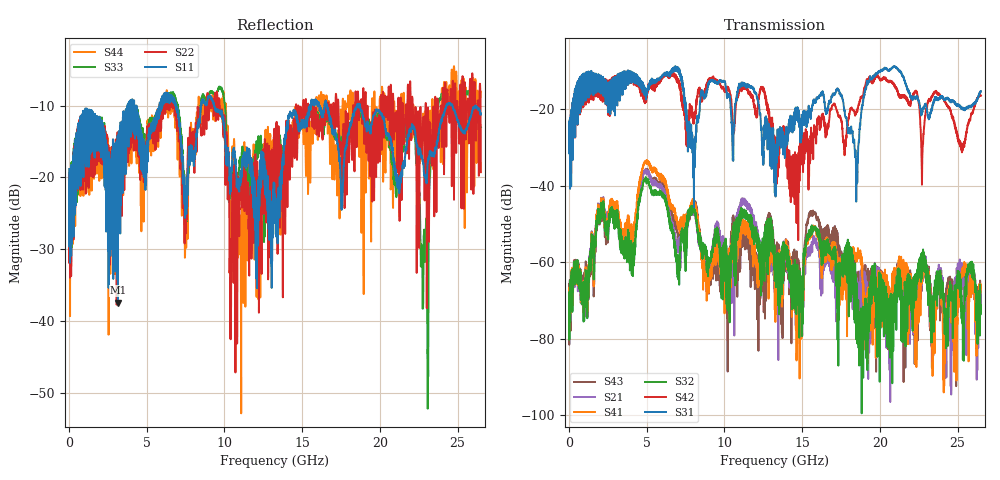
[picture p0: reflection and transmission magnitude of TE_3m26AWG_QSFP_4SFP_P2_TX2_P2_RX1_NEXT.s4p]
!Agilent Technologies,N5222A,MY51421691,A.10.00.00
!Agilent N5222A: A.10.00.00
!Date: Friday, January 30, 2015 12:35:11
!Correction: S11(Full 4 Port(1,2,3,4))
!S12(Full 4 Port(1,2,3,4))
!S13(Full 4 Port(1,2,3,4))
!S14(Full 4 Port(1,2,3,4))
!S21(Full 4 Port(1,2,3,4))
!S22(Full 4 Port(1,2,3,4))
!S23(Full 4 Port(1,2,3,4))
!S24(Full 4 Port(1,2,3,4))
!S31(Full 4 Port(1,2,3,4))
!S32(Full 4 Port(1,2,3,4))
!S33(Full 4 Port(1,2,3,4))
!S34(Full 4 Port(1,2,3,4))
!S41(Full 4 Port(1,2,3,4))
!S42(Full 4 Port(1,2,3,4))
!S43(Full 4 Port(1,2,3,4))
!S44(Full 4 Port(1,2,3,4))
!S4P File: Measurements: <S11,S12,S13,S14>,
!<S21,S22,S23,S24>,
!<S31,S32,S33,S34>,
!<S41,S42,S43,S44>:
# Hz S  dB  R 50.0
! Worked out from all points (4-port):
!   2650 points, 10 MHz to 26.5 GHz, reference 50 ohm
!   strongest paths, dB at 10 MHz, 6.63 GHz, 13.26 GHz, 19.88 GHz, 26.5 GHz:
!     S31: -24.9, -10.2, -30.2, -10.6, -15.3
!     S42: -24.8, -11.4, -27.6, -11.4, -16.5
!     S32: -67.9, -52.4, -58.5, -79.4, -71.2
!     S41: -66.7, -46.2, -58.7, -65.3, -65.8
!     S21: -67.4, -50.9, -58.9, -62.4, -69.3
!     S43: -65.6, -48.8, -58.1, -69.2, -69.2
!   lowest |S11| = -37.4 dB at 3.15 GHz (marker M1), VSWR 1.03, Z = 50.6 - j1.22 ohm
!   |S11| at or under -10 dB: start of sweep to 3.77 GHz; 9.336 GHz to 15.5 GHz (6.161 GHz wide, 49.6 % of centre); 18.72 GHz to 24.29 GHz (5.565 GHz wide, 25.9 % of centre)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
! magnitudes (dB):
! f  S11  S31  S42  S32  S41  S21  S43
! 10 MHz  -18.8  -24.9  -24.8  -67.9  -66.7  -67.4  -65.6
! 3.15 GHz  -37.4  -17.0  -16.0  -47.4  -45.2  -45.9  -46.7
! 14.32 GHz  -11.5  -22.8  -42.6  -61.7  -61.0  -60.8  -62.4
! 22 GHz  -13.6  -17.2  -18.5  -66.7  -65.6  -64.5  -66.1
! 23.01 GHz  -20.8  -20.0  -19.6  -61.2  -62.1  -63.4  -65.4
! 23.89 GHz  -12.5  -16.9  -16.5  -62.1  -67.0  -64.0  -68.4
! 26.5 GHz  -11.1  -15.3  -16.5  -71.2  -65.8  -69.3  -69.2
